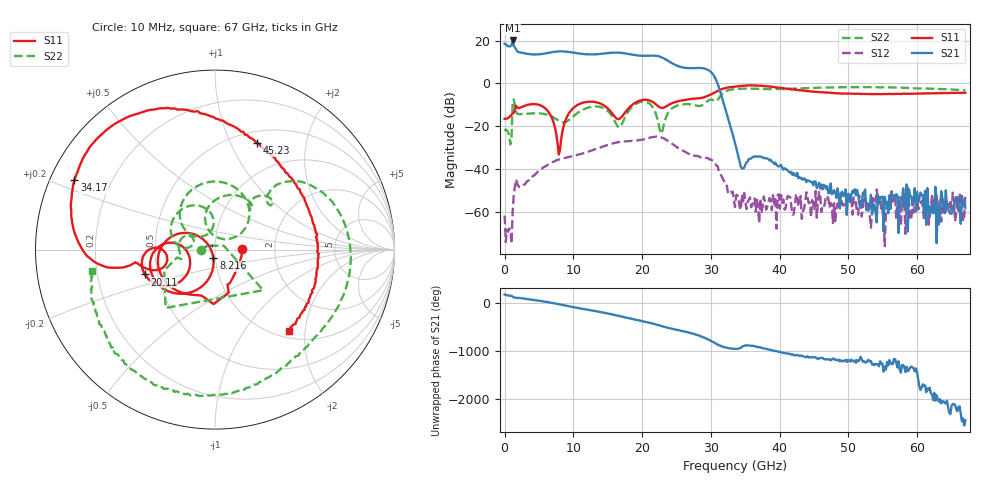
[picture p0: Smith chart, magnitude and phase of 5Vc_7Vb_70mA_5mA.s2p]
! MARKI MICROWAVE INC.
! Date:  05/05/2020
! Model Number:  APM-7099CH
! Description:  2-port Small Signal S-parameter data for APM-7099CH
! Frequency Range:  10 MHz to 67 GHz
! Port Configuration:  PORT 1: Input
!  PORT 2: Output
! Bias Condition: Vc = +5V, Vb = +7V
! APM-7099CH s2p files are only valid for small signal conditions (below -5 dBm input power)
!S2P File: Measurements: Mag<S11> Ang<S11>, Mag<S21> Ang<S21>, Mag<S12> Ang<S12>, Mag<S22> Ang<S22>!row 1
# Hz S  dB  R 50
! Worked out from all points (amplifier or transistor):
!   401 points, 10 MHz to 67 GHz, reference 50 ohm
!   highest |S21| = 20.0 dB at 1.182 GHz (marker M1)
!   |S21| within 3 dB of that: start of sweep to 1.437 GHz
!   unconditionally stable (mu >= 1): start of sweep to end of sweep
!   at 11.06 GHz: K = 3.80, MAG = 14.6 dB, |S12| = -32.8 dB
!   at 33.51 GHz: K = 1124.78, MAG = -18.6 dB, |S12| = -57.5 dB
!   at 67 GHz: K = 43734.96, MAG = -52.9 dB, |S12| = -50.9 dB
!   S11 on the Smith chart (normalised r, x): 10 MHz: 1.35, +0.00; 8.216 GHz: 0.98, -0.09; 20.11 GHz: 0.42, -0.14; 34.17 GHz: 0.07, +0.23; 45.23 GHz: 0.63, +1.26; 67 GHz: 1.14, -1.64
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1e7  -16.46 0.5  18.49 178.7  -61.47 104.7  -22.14 -177.3
1.182325e9  -13.80 -66.1  20.02 138.8  -59.63 69.4  -9.10 -40.2
1.68475e9  -10.35 -91.5  15.90 108.4  -44.63 -81.3  -13.34 -168.4
4.866775e9  -9.82 -170.4  13.54 53.0  -41.01 179.3  -13.87 169.8
8.216275e9  -26.31 -100.9  14.94 -33.1  -35.08 91.6  -17.83 156.9
9.556075e9  -12.99 -110.7  14.58 -72.0  -34.02 59.4  -16.48 175.8
1.123082e10  -9.09 -139.2  13.79 -116.4  -32.65 24.9  -12.46 166.9
1.40779e10  -9.54 -179.5  13.82 171.6  -29.60 -38.9  -11.06 118.9
1.642255e10  -16.48 -168.8  14.38 99.8  -27.38 -102.7  -19.88 106.4
1.826478e10  -10.78 -138.7  13.60 40.1  -26.81 -155.6  -11.85 139.3
2.0107e10  -7.64 -160.5  12.88 -16.3  -26.04 153.2  -8.42 92.1
2.245165e10  -10.83 -179.0  12.63 -102.0  -24.85 69.1  -19.68 35.7
2.395892e10  -9.78 -160.3  10.17 -161.1  -27.08 8.9  -12.84 101.1
2.6806e10  -7.36 -168.6  7.13 106.5  -32.76 -80.2  -9.62 55.5
2.88157e10  -6.60 -170.1  7.11 13.6  -34.30 -163.0  -9.95 52.6
2.998802e10  -5.14 -169.5  5.43 -64.3  -35.31 124.1  -7.51 42.6
3.3505e10  -1.42 160.1  -27.61 127.7  -57.53 -20.5  -2.57 8.3
3.41749e10  -1.17 153.7  -36.29 140.0  -57.06 -40.7  -2.44 -0.9
4.472582e10  -3.72 71.5  -45.87 -43.8  -54.25 48.0  -2.07 -74.9
4.522825e10  -3.89 68.7  -45.77 -49.1  -50.08 -51.0  -2.05 -77.4
5.594665e10  -4.80 8.6  -52.01 -103.6  -56.82 -136.1  -1.81 -126.4
6.7e10  -4.28 -47.6  -57.81 80.6  -50.86 -11.2  -3.14 -170.3
